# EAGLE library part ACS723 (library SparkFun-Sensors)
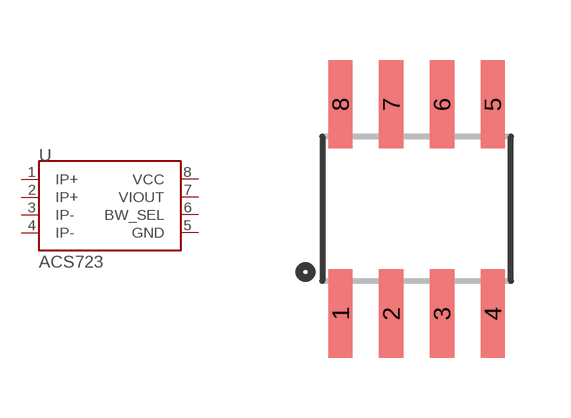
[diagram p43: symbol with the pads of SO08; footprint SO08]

Designator prefix -

## ACS723 (PART_#: ACS723ACS723LLCTR-05AB-T2; PROD_ID: IC-13872)  [SO08]
1  IP+  in
2  IP+  in
3  IP-
4  IP-
5  GND
6  BW_SEL
7  VIOUT
8  VCC

## Footprint SO08 (pad centres in mm)
Small Outline Package Fits JEDEC packages (narrow SOIC-8)
smd 0.61 x 2.21: 1 -1.905,-2.616; 2 -0.635,-2.616; 3 0.635,-2.616; 4 1.905,-2.616; 5 1.905,2.616; 6 0.635,2.616; 7 -0.635,2.616; 8 -1.905,2.616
